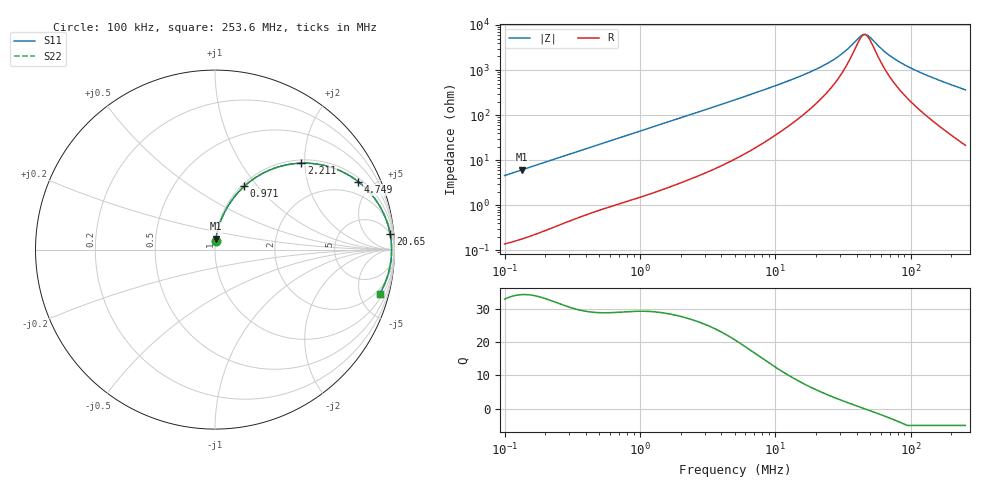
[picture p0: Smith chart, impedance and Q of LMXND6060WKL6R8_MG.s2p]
! LMXND6060WKL6R8_MG  S-PARAMETER MODEL  ( General Type )
! Model Generated by TAIYO YUDEN Corporation (http://www.ty-top.com)
! Version 1.0
! TAIYO YUDEN Control No. 191025NI43SB-FBB
! Copyright(c) 2019 TAIYO YUDEN CO.,LTD. All Rights Reserved.
! Product Description (link to TY-COMPAS)
! https://ds.yuden.co.jp/TYCOMPAS/or/detail?pn=LMXND6060WKL6R8NMG&u=M
! Products Name : Inductors
! Characteristics :
!  Inductance : 6.8 uH , SRF(min) : 30 MHz , DC Resistance(max) : 0.102 Ohm
!  Rated Current : Saturation :2000 mA , Temp Rise : 1800 mA
!  Case Size : 6.0 x 6.0 / 0.236 x 0.236 [mm/inch] , Thickness : 2 / 0.079 [mm/inch]
!  (Conditions: Temperature = 25 degC , DC Bias Current/Voltage = 0A / 0V)
! External Node Assignments :
!  1  o---GGG---o  2
! GND o---------o GND
! Frequency Range : 0.1MHz  -  253.640152MHz  [ 402 STEP ]
# MHz S RI R 50
! Freq[MHz].  S11 Real  S11 Imag  S21 Real  S21 Imag  S12 Real  S12 Imag  S22 Real  S22 Imag
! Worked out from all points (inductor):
!   401 points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, 100 kHz to 253.6 MHz, reference 50 ohm
!   read as one part in series: L = 7.27 uH near 104 kHz
!   highest Q = 34.2 at 134.2 kHz (marker M1), where L = 7.27 uH
!   self-resonance near 45.7 MHz
!   S11 on the Smith chart (normalised r, x): 100 kHz: 1.00, +0.09; 971 kHz: 1.03, +0.85; 2.211 MHz: 1.07, +1.92; 4.749 MHz: 1.19, +4.12; 20.65 MHz: 5, +21; 253.6 MHz: 1.43, -7.26
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0.1  0.00347 0.0455  0.9965 -0.0455  0.9965 -0.0455  0.00347 0.0455
0.134171  0.00551 0.0608  0.9945 -0.0608  0.9945 -0.0608  0.00551 0.0608
0.371712  0.0323 0.1607  0.9677 -0.1607  0.9677 -0.1607  0.0323 0.1607
0.630945  0.0803 0.255  0.9197 -0.255  0.9197 -0.255  0.0803 0.255
0.971009  0.1628 0.3524  0.8372 -0.3524  0.8372 -0.3524  0.1628 0.3524
1.381698  0.2746 0.4294  0.7254 -0.4294  0.7254 -0.4294  0.2746 0.4294
2.211394  0.4811 0.4816  0.5189 -0.4816  0.5189 -0.4816  0.4811 0.4816
3.146704  0.6451 0.4589  0.3549 -0.4589  0.3549 -0.4589  0.6451 0.4589
4.748729  0.7987 0.3781  0.2013 -0.3781  0.2013 -0.3781  0.7987 0.3781
5.03627  0.8159 0.3641  0.1841 -0.3641  0.1841 -0.3641  0.8159 0.3641
8.890267  0.9253 0.2293  0.0747 -0.2293  0.0747 -0.2293  0.9253 0.2293
18.72042  0.9735 0.0994  0.0265 -0.0994  0.0265 -0.0994  0.9735 0.0994
20.64754  0.9761 0.0864  0.0239 -0.0864  0.0239 -0.0864  0.9761 0.0864
29.96185  0.9821 0.0429  0.0179 -0.0429  0.0179 -0.0429  0.9821 0.0429
34.36706  0.9832 0.0286  0.0168 -0.0286  0.0168 -0.0286  0.9832 0.0286
41.80689  0.984 0.00882  0.016 -0.00882  0.016 -0.00882  0.984 0.00882
45.21578  0.984 0.00105  0.016 -0.00105  0.016 -0.00105  0.984 0.00105
49.87039  0.984 -0.00866  0.016 0.00866  0.016 0.00866  0.984 -0.00866
69.58603  0.9822 -0.0428  0.0178 0.0428  0.0178 0.0428  0.9822 -0.0428
86.32529  0.9795 -0.067  0.0205 0.067  0.0205 0.067  0.9795 -0.067
115.8234  0.9728 -0.1047  0.0272 0.1047  0.0272 0.1047  0.9728 -0.1047
253.6402  0.9172 -0.2477  0.0828 0.2477  0.0828 0.2477  0.9172 -0.2477
